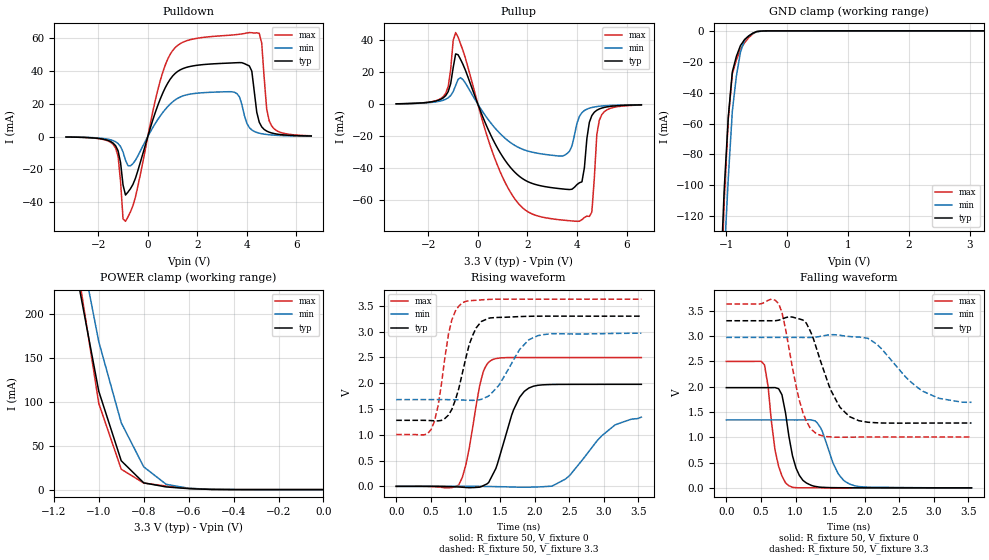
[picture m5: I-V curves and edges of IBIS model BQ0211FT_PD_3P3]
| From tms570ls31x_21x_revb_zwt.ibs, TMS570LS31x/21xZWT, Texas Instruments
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|   Model Cell BQ0211FT_PD_3P3
|BQ0211FT_PD_3P3
[Model]   BQ0211FT_PD_3P3
Model_type   I/O
Polarity   Non-Inverting
Enable   Active-Low
Vinl =  1.15
Vinh =  1.55
Cref =  15.0001pF
Rref =  101.0000M
Vref =  0V
Vmeas =  1.65
C_comp   1.2p   1.2p   1.2p
[Model Spec]
Vinl   1.15   1.02   1.28
Vinh   1.55   1.45   1.65
[Temperature Range]   25   155   -40
[Voltage Range]   3.3   2.97   3.63
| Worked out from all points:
|   slope of the pulldown table from 0 to 0.495 V, typ, clamps not added: 22 ohm
|   slope of the pullup table from 0 to 0.495 V, typ, clamps not added: 26.9 ohm
|   GND clamp passes 1 mA (typ) near -0.53 V on its own axis
|   POWER clamp passes 1 mA (typ) near -0.59 V on its own axis
|   rising waveform, R_fixture 50, V_fixture 0: 20-80 % time 279ps typ, 513ps min, 195ps max; typ from 0 V to 1.98 V
|   rising waveform, R_fixture 50, V_fixture 3.3: 20-80 % time 239ps typ, 354ps min, 183ps max; typ from 1.28 V to 3.3 V
|   falling waveform, R_fixture 50, V_fixture 0: 20-80 % time 166ps typ, 225ps min, 139ps max; typ from 1.98 V to 0 V
|   falling waveform, R_fixture 50, V_fixture 3.3: 20-80 % time 335ps typ, 536ps min, 238ps max; typ from 3.3 V to 1.28 V
[POWER_clamp]
|   voltage   I(typ)   I(min)   I(max)
-3.3V     4.054A     4.63A      4.887A
-1.1V     248.3mA    301mA      262.7mA
-1.067V   202.9mA    256.9mA    207.9mA
-1.033V   157.5mA    212.7mA    153.1mA
-1V       112.1mA    168.6mA    98.31mA
-900mV    32.89mA    76.23mA    23.26mA
-800mV    7.724mA    25.95mA    7.513mA
-700mV    3.052mA    6.046mA    4.028mA
-600mV    1.107mA    1.536mA    1.463mA
-500mV    206.8uA    377.5uA    241.6uA
0V        19.75uA    8.57uA     38.26uA
[Pulldown]
|   voltage   I(typ)   I(min)   I(max)
-3.3V     -289uA     -253.9uA   -287.1uA
-1.4V     -4mA       -2.489mA   -4.76mA
-1.2V     -8.69mA    -4.261mA   -12.05mA
-1V       -29.49mA   -9.376mA   -50.19mA
-900mV    -35.6mA    -14.42mA   -51.59mA
1V        36.78mA    21.07mA    52.28mA
3.5V      44.86mA    26.91mA    61.93mA
4.1V      42.98mA    5.455mA    63.29mA
4.6V      5.887mA    1.718mA    56.92mA
4.8V      3.323mA    1.257mA    16.92mA
5V        2.171mA    957.9uA    6.458mA
6.6V      331.3uA    239.5uA    466.8uA
[Pullup]
|   voltage   I(typ)   I(min)   I(max)
-3.3V     325.3uA    297.6uA    301.6uA
-1.4V     4.042mA    2.556mA    4.795mA
-1.2V     7.932mA    4.062mA    11.12mA
-900mV    31.45mA    11.76mA    44.76mA
1.4V      -40.91mA   -24.77mA   -56.99mA
3.4V      -52.76mA   -32.29mA   -72.18mA
4V        -50.08mA   -11.8mA    -72.98mA
4.2V      -48.37mA   -5.201mA   -71.98mA
4.6V      -7.019mA   -1.989mA   -67.23mA
4.8V      -3.708mA   -1.414mA   -19.03mA
5V        -2.349mA   -1.055mA   -6.475mA
6.6V      -340.9uA   -258.1uA   -448.7uA
[GND_clamp]
|   voltage   I(typ)   I(min)   I(max)
-3.3V     -3.25A     -2.875A    -4.945A
-1.1V     -166.9mA   -205mA     -187mA
-1.033V   -102.8mA   -146.7mA   -110.1mA
-966.7mV  -55.96mA   -95.69mA   -57.02mA
-900mV    -26.55mA   -52.03mA   -27.8mA
-833.3mV  -16.5mA    -29.28mA   -18.78mA
-766.7mV  -9.547mA   -13.91mA   -12.08mA
-700mV    -5.701mA   -5.927mA   -7.726mA
-566.7mV  -1.578mA   -1.635mA   -2.073mA
-500mV    -412.7uA   -599.4uA   -476.8uA
-366.7mV  -26.33uA   -63.11uA   -29.79uA
3.233V    19.75uA    12.65uA    38.26uA
[Ramp]
| variable   typ   min   max
dV/dt_f   1.260445/0.3439348n  0.8122765/0.5595231n   1.637936/0.245536n
dV/dt_r   1.203143/0.2803609n  0.8163021/0.5195282n   1.517414/0.1979105n
R_load = 50
[Rising Waveform]
R_fixture = 50
V_fixture = 0
V_fixture_min = 0
V_fixture_max = 0
|   time   V(typ)   V(min)   V(max)
0s        -6.029uV   -2.875uV   -3.536uV
904ps     -12.68mV   195.4uV    25.98mV
1.008ns   -22.58mV   252.9uV    423.4mV
1.26ns    14.21mV    -1.902mV   2.229V
1.388ns   208.7mV    -4.422mV   2.455V
1.696ns   1.482V     -13.96mV   2.497V
1.916ns   1.905V     -16.81mV   2.497V
2.444ns   1.977V     139.3mV    2.496V
3.164ns   1.978V     1.192V     2.497V
3.544ns   1.978V     1.341V     2.497V
[Rising Waveform]
R_fixture = 50
V_fixture = 3.3
V_fixture_min = 2.97
V_fixture_max = 3.63
|   time   V(typ)   V(min)   V(max)
0s        1.28V      1.682V     1.005V
504ps     1.275V     1.682V     1.1V
604ps     1.269V     1.682V     1.554V
804ps     1.492V     1.68V      3.228V
956ps     2.194V     1.674V     3.561V
1.156ns   3.072V     1.671V     3.608V
1.336ns   3.258V     1.751V     3.624V
1.784ns   3.292V     2.654V     3.63V
2.048ns   3.299V     2.921V     3.629V
3.544ns   3.3V       2.969V     3.629V
[Falling Waveform]
R_fixture = 50
V_fixture = 0
V_fixture_min = 0
V_fixture_max = 0
|   time   V(typ)   V(min)   V(max)
0s        1.979V     1.342V     2.497V
552ps     1.978V     1.342V     2.428V
704ps     1.98V      1.342V     746.7mV
804ps     1.837V     1.342V     236.2mV
904ps     1.022V     1.342V     42.92mV
1.056ns   245.4mV    1.341V     423.9uV
1.26ns    35.41mV    1.33V      751.9uV
1.616ns   3.024mV    283.3mV    488.8uV
1.784ns   1.601mV    74.26mV    492.9uV
3.544ns   284.4uV    562.2uV    19.92uV
[Falling Waveform]
R_fixture = 50
V_fixture = 3.3
V_fixture_min = 2.97
V_fixture_max = 3.63
|   time   V(typ)   V(min)   V(max)
0s        3.3V       2.97V      3.63V
756ps     3.31V      2.97V      3.639V
804ps     3.332V     2.97V      3.465V
1.108ns   3.313V     2.97V      1.484V
1.312ns   2.716V     2.981V     1.06V
1.516ns   1.914V     3.023V     1.006V
1.784ns   1.405V     2.987V     1.001V
2.18ns    1.285V     2.831V     1.005V
2.84ns    1.279V     1.908V     1.005V
3.544ns   1.28V      1.689V     1.005V
